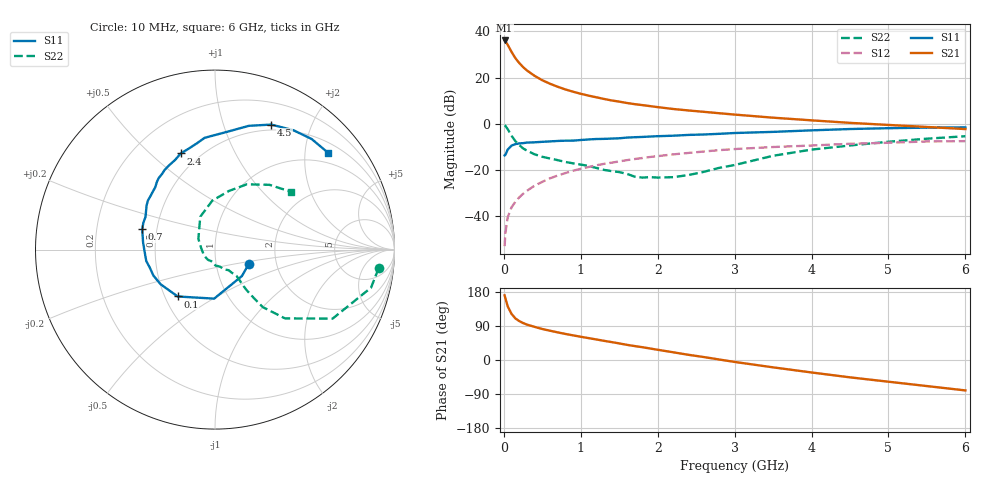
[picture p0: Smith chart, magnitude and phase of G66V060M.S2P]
! SIEMENS Small Signal Semiconductors
! BFG193
! Si NPN RF Bipolar Junction Transistor in SOT223
! VCE = 6 V  IC = 60 mA
! Common Emitter S-Parameters:  August  1996
# GHz  S  MA  R  50
!  f  S11  S21  S12  S22
! GHz  MAG  ANG  MAG  ANG  MAG  ANG  MAG  ANG
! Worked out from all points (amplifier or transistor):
!   36 points, 10 MHz to 6 GHz, reference 50 ohm
!   highest |S21| = 36.1 dB at 10 MHz (marker M1)
!   |S21| within 3 dB of that: start of sweep to 68.2 MHz
!   unconditionally stable (mu >= 1): 427.5 MHz to 2.376 GHz
!   at 250 MHz: K = 0.93, MSG = 27.5 dB, |S12| = -30.5 dB
!   at 1.4 GHz: K = 1.04, MAG = 12.2 dB, |S12| = -16.9 dB
!   at 6 GHz: K = 0.89, MSG = 2.6 dB, |S12| = -7.6 dB
!   S11 on the Smith chart (normalised r, x): 10 MHz: 1.44, -0.25; 100 MHz: 0.58, -0.34; 700 MHz: 0.41, +0.11; 2.4 GHz: 0.40, +0.63; 4.5 GHz: 0.44, +1.46; 6 GHz: 0.73, +2.52
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0.01  0.2046 -23.6  63.61 170.7  0.0022 89.7  0.9176 -6.5
0.02  0.2103 -44.5  61.05 162.8  0.0042 80.5  0.8949 -13.7
0.05  0.2732 -91.0  51.25 141.6  0.0093 72.9  0.7598 -30.4
0.1  0.3338 -128.5  35.93 121.7  0.0153 67.8  0.5469 -44.5
0.15  0.3596 -147.6  26.28 109.6  0.0202 66.8  0.4164 -50.3
0.2  0.3724 -157.2  20.69 102.8  0.0252 69.2  0.3434 -51.3
0.25  0.3771 -164.7  16.84 97.5  0.03 69.6  0.2901 -52.0
0.3  0.3881 -170.5  14.24 93.5  0.0349 70.7  0.2603 -52.0
0.4  0.3932 -179.0  10.86 87.4  0.0451 70.4  0.2158 -51.2
0.5  0.4031 174.0  8.714 81.8  0.0546 69.2  0.1908 -50.7
0.6  0.4112 168.8  7.322 77.3  0.0651 68.1  0.1752 -51.7
0.7  0.4209 164.3  6.303 72.9  0.0748 66.9  0.1614 -53.7
0.9  0.4276 155.0  4.917 65.0  0.0951 63.2  0.1375 -56.6
1.1  0.4536 147.2  4.048 57.8  0.1144 59.8  0.1206 -65.5
1.3  0.4667 140.5  3.434 50.7  0.1339 55.7  0.0994 -73.3
1.6  0.4978 130.5  2.8 40.0  0.1616 48.8  0.0812 -93.7
2.2  0.5466 114.0  2.078 20.4  0.2152 35.1  0.069 -157.1
2.4  0.5688 109.6  1.928 13.7  0.2313 30.9  0.0766 175.0
3.5  0.6621 83.6  1.345 -19.4  0.3108 3.9  0.2008 114.1
4.5  0.7637 65.8  1.039 -45.8  0.3656 -16.1  0.3355 76.7
5.5  0.8184 48.8  0.846 -68.8  0.4109 -39.4  0.4713 50.0
6  0.8293 40.6  0.762 -80.3  0.4173 -52.8  0.5332 37.1
